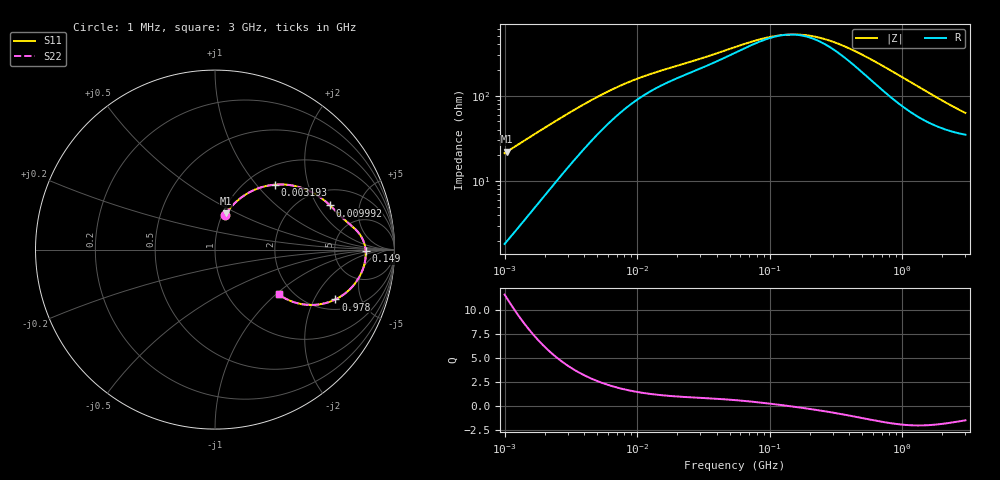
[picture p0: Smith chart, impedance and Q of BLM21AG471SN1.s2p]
! BLM21AG471SN1
# Hz S RI R 50
!Freq.(Hz) S11(Real) S11(Imag) S21(Real) S21(Imag) S12(Real) S12(Imag) S22(Real) S22(Imag)
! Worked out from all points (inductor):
!   401 points, 1 MHz to 3 GHz, reference 50 ohm
!   read as one part in series: L = 3.35 uH near 1.041 MHz
!   highest Q = 11.2 at 1.041 MHz (marker M1), where L = 3.36 uH
!   self-resonance near 137.3 MHz
!   S11 on the Smith chart (normalised r, x): 1 MHz: 1.04, +0.42; 3.193 MHz: 1.32, +1.26; 9.992 MHz: 2.79, +2.60; 149 MHz: 11, -1; 978 MHz: 2.55, -2.99; 3 GHz: 1.70, -1.04
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1000000  0.0585 0.1954  0.9415 -0.1954  0.9415 -0.1954  0.0585 0.1954
1040844  0.0628 0.2021  0.9372 -0.2021  0.9372 -0.2021  0.0628 0.2021
1786863  0.1564 0.2975  0.8436 -0.2975  0.8436 -0.2975  0.1564 0.2975
2461366  0.2472 0.3435  0.7528 -0.3435  0.7528 -0.3435  0.2472 0.3435
3192880  0.3356 0.3619  0.6644 -0.3619  0.6644 -0.3619  0.3356 0.3619
3823119  0.399 0.3615  0.601 -0.3615  0.601 -0.3615  0.399 0.3615
6180806  0.5467 0.316  0.4533 -0.316  0.4533 -0.316  0.5467 0.316
9992459  0.6414 0.246  0.3586 -0.246  0.3586 -0.246  0.6414 0.246
1.461624e7  0.688 0.1992  0.312 -0.1992  0.312 -0.1992  0.688 0.1992
5.477226e7  0.8024 0.0905  0.1976 -0.0905  0.1976 -0.0905  0.8024 0.0905
9.787053e7  0.8316 0.0349  0.1684 -0.0349  0.1684 -0.0349  0.8316 0.0349
1.49005e8  0.8395 -0.00873  0.1605 0.00873  0.1605 0.00873  0.8395 -0.00873
2.094008e8  0.8386 -0.047  0.1614 0.047  0.1614 0.047  0.8386 -0.047
2.662515e8  0.8335 -0.0767  0.1665 0.0767  0.1665 0.0767  0.8335 -0.0767
3.523638e8  0.8215 -0.1155  0.1785 0.1155  0.1785 0.1155  0.8215 -0.1155
5.473095e8  0.7823 -0.1858  0.2177 0.1858  0.2177 0.1858  0.7823 -0.1858
8.005644e8  0.7181 -0.2492  0.2819 0.2492  0.2819 0.2492  0.7181 -0.2492
9.779672e8  0.6705 -0.2778  0.3295 0.2778  0.3295 0.2778  0.6705 -0.2778
1.268618e9  0.5965 -0.3026  0.4035 0.3026  0.4035 0.3026  0.5965 -0.3026
1.645649e9  0.5155 -0.3078  0.4845 0.3078  0.4845 0.3078  0.5155 -0.3078
2.312676e9  0.4161 -0.2841  0.5839 0.2841  0.5839 0.2841  0.4161 -0.2841
3e9  0.3552 -0.2497  0.6448 0.2497  0.6448 0.2497  0.3552 -0.2497
